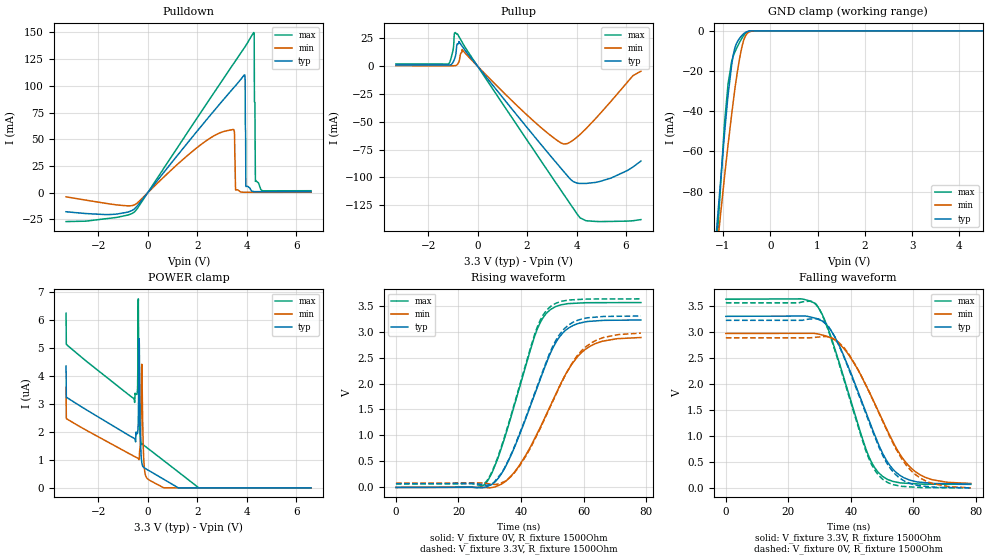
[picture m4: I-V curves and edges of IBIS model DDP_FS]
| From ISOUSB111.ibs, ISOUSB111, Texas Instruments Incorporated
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[Model]   DDP_FS
Model_type   I/O
Polarity   Non-Inverting
Enable   Active-Low
Vinl = 0.8
Vinh = 2
Vmeas = 1.65
Vref = 1.65
Cref = 7pF
Rref = 15000
|   typ   min   max
C_comp   8pF   5pF   10pF
[Voltage Range]   3.3   2.97   3.63
[Temperature Range]   27   150   -40
[Pullup Reference]   3.3   2.97   3.63
[Pulldown Reference]   -0   0   0
[Power Clamp Reference]   3.3   2.97   3.63
[GND Clamp Reference]   0   0   0
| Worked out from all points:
|   slope of the pulldown table from 0 to 0.495 V, typ, clamps not added: 34.2 ohm
|   slope of the pullup table from 0 to 0.495 V, typ, clamps not added: 35.8 ohm
|   GND clamp passes 1 mA (typ) near -0.54 V on its own axis
|   falling waveform, V_fixture 3.3V, R_fixture 1500Ohm: 20-80 % time 12.8ns typ, 14.5ns min, 11.1ns max; typ from 3.3 V to 0.073 V
|   rising waveform, V_fixture 0V, R_fixture 1500Ohm: 20-80 % time 12.4ns typ, 14.5ns min, 10.6ns max; typ from 0 V to 3.22 V
|   rising waveform, V_fixture 3.3V, R_fixture 1500Ohm: 20-80 % time 12.3ns typ, 14.2ns min, 10.5ns max; typ from 0.073 V to 3.3 V
|   falling waveform, V_fixture 0V, R_fixture 1500Ohm: 20-80 % time 12.7ns typ, 14.1ns min, 11ns max; typ from 3.22 V to 0 V
[Pulldown]
|   Voltage   I(typ)   I(min)   I(max)
-3.3V     -17.81mA   -3.85mA    -26.98mA
-537.9mV  -15.2mA    -11.4mA    -18.05mA
3.452V    97.57mA    59.13mA    120.1mA
3.551V    100.2mA    2.568mA    123.5mA
3.907V    110.2mA    416.5uA    135.6mA
3.937V    106.3mA    416.5uA    136.7mA
3.967V    5.859mA    416.5uA    137.7mA
4.283V    1.074mA    416.6uA    149.8mA
4.303V    991.3uA    416.6uA    149mA
4.313V    991.1uA    416.6uA    85.12mA
4.353V    991.5uA    416.7uA    10.62mA
6.6V      1.044mA    452.8uA    1.864mA
[GND Clamp]
|   Voltage   I(typ)   I(min)   I(max)
-3.3V     -1.286A    -1.121A    -1.579A
-1.3V     -145.3mA   -147.2mA   -170.6mA
-973.5mV  -52.59mA   -73.66mA   -47.68mA
-894.3mV  -32.06mA   -56.81mA   -26.49mA
-815.1mV  -16.5mA    -41.06mA   -14.88mA
-785.4mV  -12.23mA   -35.46mA   -12.65mA
-735.9mV  -7.575mA   -26.62mA   -9.853mA
-627mV    -3.033mA   -10.97mA   -4.745mA
-567.6mV  -1.539mA   -5.066mA   -2.489mA
-498.3mV  -471.8uA   -1.571mA   -746.6uA
-260.7mV  0A         -5.306uA   0A
6.6V      0A         0A         0A
[Pullup]
|   Voltage   I(typ)   I(min)   I(max)
-3.3V     1.143mA    463.2uA    2.099mA
-1.181V   1.062mA    442.5uA    1.996mA
-993.3mV  3.496mA    442.2uA    14.19mA
-933.9mV  6.482mA    535.1uA    29.92mA
-815.1mV  20.26mA    1.636mA    29.12mA
-627mV    18.09mA    14.99mA    21.7mA
1.957V    -54.04mA   -43.09mA   -65.14mA
3.491V    -95.04mA   -70.01mA   -115.7mA
3.868V    -103.9mA   -66.43mA   -128mA
4.382V    -105.5mA   -56.22mA   -139.1mA
5.392V    -100.7mA   -31.56mA   -139.7mA
6.6V      -85.38mA   -4.479mA   -138.1mA
[POWER Clamp]
|   Voltage   I(typ)   I(min)   I(max)
-3.3V     4.356uA    3.599uA    6.245uA
-3.29V    3.24uA     2.478uA    5.13uA
-528mV    1.759uA    1.119uA    3.053uA
-409.2mV  1.963uA    1.064uA    3.57uA
-379.5mV  2.509uA    1.044uA    6.758uA
-349.8mV  5.335uA    1.011uA    3.278uA
-300.3mV  1.978uA    1.538uA    1.841uA
-250.8mV  984.9nA    4.227uA    1.559uA
-171.6mV  741.8nA    1.249uA    1.531uA
-62.7mV   674.2nA    385.9nA    1.457uA
2.056V    0A         0A         4.445nA
6.6V      0A         0A         0A
[Ramp]
R_load = 1500
|   typ   min   max
dV/dt_r   1.93339/1.2374e-08   1.73122/1.44206e-08   2.13488/1.05473e-08
dV/dt_f   1.93542/1.282e-08   1.73113/1.44351e-08   2.13691/1.10541e-08
[Falling Waveform]
V_fixture = 3.3V
V_fixture_min = 2.97V
V_fixture_max = 3.63V
R_fixture = 1500Ohm
C_fixture = 0F
|   Time   V(typ)   V(min)   V(max)
0s        3.299V     2.969V     3.629V
28.18ns   3.269V     2.972V     3.559V
31.52ns   3.176V     2.93V      3.243V
35.96ns   2.774V     2.79V      2.466V
44.98ns   1.428V     1.953V     717.8mV
48.64ns   866.3mV    1.491V     304.5mV
53.85ns   331.6mV    836.3mV    118.6mV
60.64ns   121mV      310mV      78.34mV
66.13ns   86.39mV    154.8mV    70.52mV
78.33ns   73.35mV    83.9mV     67.4mV
[Rising Waveform]
V_fixture = 0V
V_fixture_min = 0V
V_fixture_max = 0V
R_fixture = 1500Ohm
C_fixture = 0F
|   Time   V(typ)   V(min)   V(max)
0s        -34.15uV   -42.85uV   -28.52uV
28.18ns   733.5uV    -529.6uV   47.19mV
30.77ns   61.93mV    -1.109mV   288.8mV
35.96ns   510.8mV    166.9mV    1.189V
44.25ns   1.771V     927.5mV    2.891V
47.96ns   2.37V      1.388V     3.341V
53.29ns   2.969V     2.065V     3.519V
60.64ns   3.187V     2.66V      3.555V
66.13ns   3.214V     2.815V     3.556V
78.33ns   3.222V     2.885V     3.558V
[Rising Waveform]
V_fixture = 3.3V
V_fixture_min = 2.97V
V_fixture_max = 3.63V
R_fixture = 1500Ohm
C_fixture = 0F
|   Time   V(typ)   V(min)   V(max)
0s        73.35mV    83.9mV     67.4mV
28.18ns   49.36mV    81.55mV    69.35mV
30.77ns   77.31mV    63.43mV    311.4mV
34.85ns   389.1mV    118.5mV    999.2mV
44.34ns   1.81V      918.4mV    2.944V
48.15ns   2.427V     1.396V     3.408V
53.29ns   3.018V     2.058V     3.586V
60.19ns   3.251V     2.678V     3.622V
66.52ns   3.291V     2.888V     3.627V
78.33ns   3.299V     2.969V     3.629V
[Falling Waveform]
|Gnd
V_fixture = 0V
V_fixture_min = 0V
V_fixture_max = 0V
R_fixture = 1500Ohm
C_fixture = 0F
|   Time   V(typ)   V(min)   V(max)
0s        3.222V     2.885V     3.558V
28.18ns   3.252V     2.893V     3.567V
32.92ns   3.095V     2.9V       3.001V
37.88ns   2.501V     2.691V     2.057V
44.72ns   1.437V     1.982V     722.9mV
48.74ns   817.9mV    1.466V     248.5mV
53.85ns   282mV      810.6mV    57.69mV
60.64ns   56.6mV     254.8mV    12.31mV
66.52ns   14.49mV    76.61mV    3.507mV
78.33ns   -34.15uV   -42.85uV   -28.52uV
